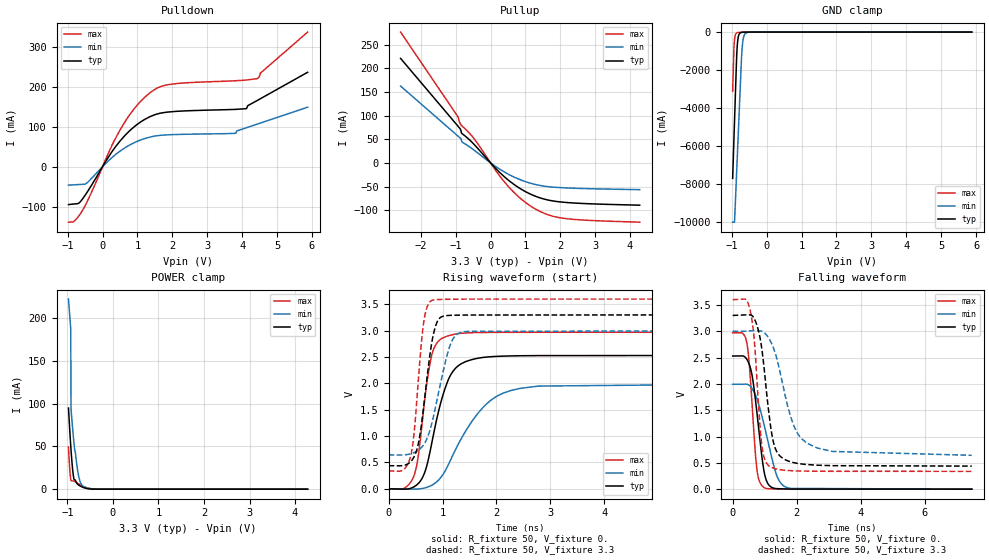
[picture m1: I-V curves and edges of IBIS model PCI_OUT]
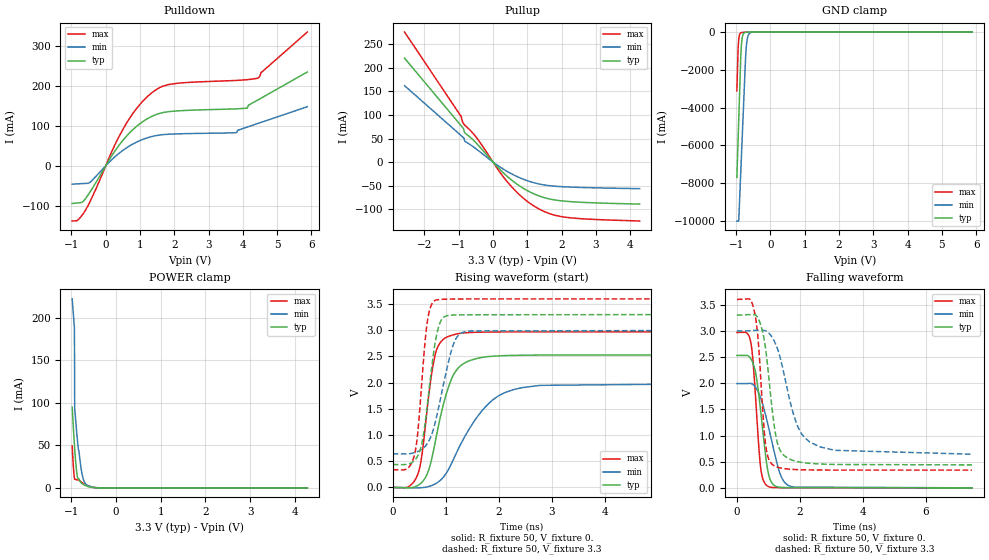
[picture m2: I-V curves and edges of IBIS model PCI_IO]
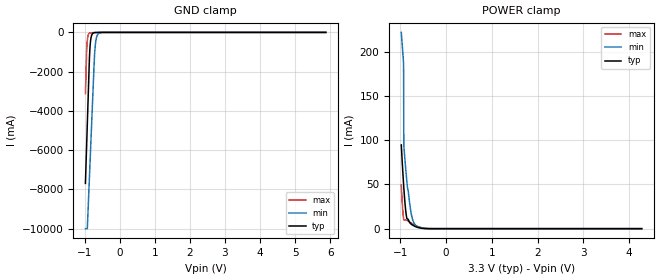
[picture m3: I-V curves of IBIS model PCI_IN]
|   IBIS Model for tsi381
[IBIS Ver]   3.2
[Disclaimer] THIS IBIS MODEL HAS BEEN CREATED BY THE SIGNAL
   INTEGRITY SOFTWARE SPICE-TO-IBIS PROCESS.
   THESE IBIS MODELS ARE PROVIDED "AS IS" WITH NO
   WARRANTY WHATSOEVER AND SIGNAL INTEGRITY SOFTWARE
   SPECIFICALLY DISCLAIMS ANY IMPLIED WARRANTIES OF
   MERCHANTABILITY, FITNESS FOR A PARTICULAR PURPOSE,
   OR AGAINST INFRINGEMENT.
[File Name]   tsi381_pbga.ibs
[File Rev]   1.4
[Date]   07/29/2009
[Notes]
   Revision History
   Rev 1.0
   - 5/30/07 Inital Release. IBIS model generated from
   SPICE model extraction. TSC
   Rev 1.3
   - 11/13/08  Updated 'model_name' definitions. IGT
   Rev 1.4
   - updated with IDT formatting
[Component] tsi381
[Manufacturer] IDT
|   typ   min   max
[Package]
R_pkg   354m   244m   481m
L_pkg   4.50nH   2.81nH   7.01nH
C_pkg   0.86pF   0.64pF   1.33pF
[Pin]  signal_name   model_name   R_pin   L_pin   C_pin
C9   GPIO[0]   NC   299.8m   3.7nh   0.83pf
A10   GPIO[1]   NC   274.4m   3.5nh   0.76pf
B10   GPIO[2]   NC   247.9m   3.3nh   0.64pf
A11   GPIO[3]   NC   287.0m   3.6nh   0.79pf
M2   JTAG_TCK   JTAG_IN   366.2m   4.4nh   0.83pf
L3   JTAG_TDI   JTAG_IN   382.4m   4.9nh   0.94pf
L1   JTAG_TDO   JTAG_OUT   371.7m   4.5nh   0.76pf
M12   JTAG_TMS   JTAG_IN   393.2m   4.5nh   0.85pf
L10   JTAG_TRSTn   JTAG_IN   410.4m   5.3nh   0.96pf
D3   PCI_AD[0]   PCI_IO   398.2m   5.4nh   0.99pf
C1   PCI_AD[1]   PCI_IO   344.1m   4.1nh   0.77pf
F4   PCI_AD[10]   PCI_IO   402.7m   5.8nh   1.06pf
G1   PCI_AD[11]   PCI_IO   310.8m   3.7nh   0.64pf
G2   PCI_AD[12]   PCI_IO   330.2m   4.0nh   0.77pf
G3   PCI_AD[13]   PCI_IO   375.2m   4.9nh   0.90pf
H1   PCI_AD[14]   PCI_IO   311.3m   3.8nh   0.65pf
H2   PCI_AD[15]   PCI_IO   355.7m   4.5nh   0.82pf
J5   PCI_AD[16]   PCI_IO   481.4m   6.8nh   1.29pf
L6   PCI_AD[17]   PCI_IO   343.6m   4.4nh   0.79pf
M6   PCI_AD[18]   PCI_IO   304.3m   3.8nh   0.66pf
K6   PCI_AD[19]   PCI_IO   371.5m   5.1nh   0.92pf
D1   PCI_AD[2]   PCI_IO   330.9m   3.9nh   0.72pf
J6   PCI_AD[20]   PCI_IO   386.3m   5.7nh   1.04pf
M7   PCI_AD[21]   PCI_IO   301.3m   3.7nh   0.65pf
L7   PCI_AD[22]   PCI_IO   326.6m   4.1nh   0.77pf
K7   PCI_AD[23]   PCI_IO   373.6m   4.9nh   0.92pf
L8   PCI_AD[24]   PCI_IO   357.1m   4.4nh   0.81pf
K8   PCI_AD[25]   PCI_IO   437.6m   5.8nh   1.12pf
M9   PCI_AD[26]   PCI_IO   323.3m   3.9nh   0.69pf
L9   PCI_AD[27]   PCI_IO   357.9m   4.5nh   0.84pf
K12   PCI_AD[28]   PCI_IO   346.8m   4.1nh   0.79pf
J11   PCI_AD[29]   PCI_IO   377.8m   4.7nh   0.93pf
D2   PCI_AD[3]   PCI_IO   353.3m   4.5nh   0.85pf
J12   PCI_AD[30]   PCI_IO   324.4m   4.0nh   0.74pf
J10   PCI_AD[31]   PCI_IO   436.5m   5.9nh   1.16pf
E1   PCI_AD[4]   PCI_IO   309.0m   3.7nh   0.67pf
E2   PCI_AD[5]   PCI_IO   352.5m   4.6nh   0.82pf
E3   PCI_AD[6]   PCI_IO   368.0m   5.0nh   0.94pf
E4   PCI_AD[7]   PCI_IO   480.4m   7.0nh   1.32pf
F2   PCI_AD[8]   PCI_IO   343.3m   4.2nh   0.79pf
F3   PCI_AD[9]   PCI_IO   363.1m   4.8nh   0.91pf
F1   PCI_CBEn[0]   PCI_IO   303.6m   3.7nh   0.65pf
H3   PCI_CBEn[1]   PCI_IO   392.2m   5.0nh   0.94pf
K5   PCI_CBEn[2]   PCI_IO   406.7m   5.4nh   1.06pf
M8   PCI_CBEn[3]   PCI_IO   309.0m   3.8nh   0.66pf
D12   PCI_CLK   PCI_IN   328.4m   3.9nh   0.67pf
H10   PCI_CLKO[0]   PCI_OUT   407.4m   5.6nh   1.09pf
C2   PCI_CLKO[1]   PCI_OUT   408.8m   5.2nh   0.95pf
K4   PCI_DEVSELn   PCI_IO   467.5m   6.4nh   1.28pf
M5   PCI_FRAMEn   PCI_IO   317.2m   3.8nh   0.68pf
G10   PCI_GNTn[0]   PCI_IO   377.6m   4.9nh   1.01pf
G9   PCI_GNTn[1]   PCI_OUT   404.4m   5.5nh   1.09pf
F11   PCI_GNTn[2]   PCI_OUT   346.6m   4.4nh   0.82pf
E11   PCI_GNTn[3]   PCI_OUT   340.9m   4.1nh   0.79pf
E12   PCI_INTAn   PCI_IN   321.7m   4.0nh   0.66pf
E9   PCI_INTBn   PCI_IN   395.4m   5.5nh   1.06pf
D11   PCI_INTCn   PCI_IN   380.1m   4.7nh   0.82pf
E10   PCI_INTDn   PCI_IN   390.8m   5.0nh   0.93pf
L5   PCI_IRDYn   PCI_IO   351.2m   4.5nh   0.87pf
M3   PCI_LOCKn   PCI_OUT   333.8m   4.2nh   0.69pf
D10   PCI_M66EN   PCI_IN   420.4m   5.6nh   0.97pf
J1   PCI_PAR   PCI_IO   328.0m   4.0nh   0.66pf
J3   PCI_PERRn   PCI_IO   436.6m   5.7nh   1.06pf
H12   PCI_PMEn   PCI_IN   326.8m   3.9nh   0.74pf
G11   PCI_REQn[0]   PCI_IO   348.8m   4.3nh   0.85pf
H9   PCI_REQn[1]   PCI_IN   420.8m   6.1nh   1.09pf
G12   PCI_REQn[2]   PCI_IN   305.3m   3.7nh   0.68pf
H11   PCI_REQn[3]   PCI_IN   335.4m   4.3nh   0.81pf
F10   PCI_RSTn   PCI_OUT   366.0m   4.9nh   0.90pf
J2   PCI_SERRn   PCI_IO   376.6m   4.8nh   0.83pf
L4   PCI_STOPn   PCI_IO   385.4m   4.9nh   0.95pf
M4   PCI_TRDYn   PCI_IO   326.3m   3.9nh   0.74pf
B12   PCIE_PERSTn   NC   347.3m   4.3nh   0.66pf
B6   PCIE_REFCLK_n   NC   339.4m   4.2nh   1.02pf
A6   PCIE_REFCLK_p   NC   341.4m   4.1nh   1.01pf
B7   PCIE_RXD_n   NC   253.1m   3.1nh   0.75pf
A8   PCIE_RXD_p   NC   266.3m   3.4nh   0.79pf
A4   PCIE_TXD_n   NC   249.7m   3.3nh   0.69pf
B5   PCIE_TXD_p   NC   244.8m   3.0nh   0.69pf
K11   PWRUP_EN_ARB   GEN33_IN   407.8m   5.1nh   1.04pf
M1   PWRUP_PLL_BYPASS   GEN33_IN   410.2m   4.8nh   0.93pf
B2   SR_CLK   NC   418.6m   5.1nh   0.96pf
C4   SR_CSn   NC   412.7m   5.5nh   1.33pf
A2   SR_DIN   NC   308.5m   3.8nh   0.87pf
A1   SR_DOUT   NC   366.1m   4.5nh   0.78pf
C8   TEST_BCE   NC   313.4m   4.3nh   0.96pf
B1   TEST_BIDR_CTL   NC   371.0m   4.4nh   0.80pf
A3   TEST_ON   NC   332.2m   4.3nh   0.93pf
M11   TEST_SPARE[0]   NC   371.4m   4.4nh   0.79pf
D8   TEST_SPARE[1]   NC   252.7m   2.8nh   0.70pf
K1   TEST_SPARE[2]   NC   349.1m   4.3nh   0.71pf
C10   VDD   POWER
D4   VDD   POWER
F6   VDD   POWER
F8   VDD   POWER
G6   VDD   POWER
G7   VDD   POWER
J9   VDD   POWER
K3   VDD   POWER
B3   VDD_PCI   POWER
B11   VDD_PCI   POWER
F9   VDD_PCI   POWER
G4   VDD_PCI   POWER
H5   VDD_PCI   POWER
H8   VDD_PCI   POWER
J7   VDD_PCI   POWER
L2   VDD_PCI   POWER
M10   VDD_PCI   POWER
A5   VDD_PCIE   POWER
A7   VDD_PCIE   POWER
D5   VDD_PCIE   POWER
E5   VDDA_PCIE   POWER
E7   VDDA_PLL   POWER
F5   VIO_PCI   POWER
G8   VIO_PCI   POWER
H6   VIO_PCI   POWER
B8   VSS   GND
B4   VSS   GND
C6   VSS   GND
C5   VSS   GND
D9   VSS   GND
D7   VSS   GND
D6   VSS   GND
E6   VSS   GND
F7   VSS   GND
G5   VSS   GND
H7   VSS   GND
H4   VSS   GND
A12   VSS_IO   GND
C11   VSS_IO   GND
C3   VSS_IO   GND
F12   VSS_IO   GND
J8   VSS_IO   GND
J4   VSS_IO   GND
K10   VSS_IO   GND
K2   VSS_IO   GND
C7   VSSA_PLL   GND
| Models and submodels in the file (6): PCI_OUT (Output), PCI_IO (I/O), PCI_IN (Input), JTAG_IN (Input), JTAG_OUT (Output), GEN33_IN (Input)
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[Model]   PCI_OUT
Model_type  Output
C_comp 4.536p 4.202p 4.874p
Polarity   Non-Inverting
Enable   Active-High
Vmeas =   1.32V
Cref =   10pF
Rref =   50
Vref=   0.0V
[Temperature Range]   27.0   125.0   -40.0
[Voltage Range] 3.3 3. 3.6
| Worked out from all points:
|   slope of the pulldown table from 0 to 0.495 V, typ, clamps not added: 7.81 ohm
|   slope of the pullup table from 0 to 0.495 V, typ, clamps not added: 13.9 ohm
|   GND clamp passes 1 mA (typ) near -0.58 V on its own axis
|   POWER clamp passes 1 mA (typ) near -0.59 V on its own axis
|   rising waveform, R_fixture 50, V_fixture 0.: 20-80 % time 365ps typ, 723ps min, 222ps max; typ from 0 V to 2.53 V
|   rising waveform, R_fixture 50, V_fixture 3.3: 20-80 % time 214ps typ, 317ps min, 159ps max; typ from 0.438 V to 3.3 V
|   falling waveform, R_fixture 50, V_fixture 0.: 20-80 % time 295ps typ, 484ps min, 203ps max; typ from 2.53 V to 0 V
|   falling waveform, R_fixture 50, V_fixture 3.3: 20-80 % time 338ps typ, 623ps min, 226ps max; typ from 3.3 V to 0.438 V
[Pulldown]
-976.9mV  -94.66mA   -46.06mA   -138.7mA
-817.5mV  -93.23mA   -45.29mA   -136.5mA
-595.7mV  -83.14mA   -44.21mA   -112.2mA
-429.3mV  -61.97mA   -39.17mA   -84.92mA
492.7mV   63.11mA    38.33mA    90.31mA
936.3mV   101.8mA    61.1mA     147.9mA
1.352V    124.6mA    73.73mA    184.1mA
1.851V    136.3mA    79.48mA    204.5mA
3.82V     143.1mA    83.35mA    214.6mA
4.125V    144.9mA    97.25mA    216.4mA
4.43V     165.1mA    106.2mA    220mA
5.879V    235.8mA    148.6mA    336.1mA
[Pullup]
-2.579V   220.8mA    162.3mA    276.3mA
-929mV    77.21mA    56.24mA    96.97mA
-887.4mV  73.58mA    53.57mA    85.73mA
-838.9mV  65.18mA    49.35mA    79.56mA
-818.1mV  61.78mA    43.99mA    77.84mA
-471.5mV  38.99mA    26.83mA    51.07mA
277.2mV   -21.28mA   -14.01mA   -29.14mA
623.8mV   -42.97mA   -28.22mA   -58.92mA
942.6mV   -58.4mA    -38.19mA   -80.33mA
1.442V    -74.52mA   -48.11mA   -103.5mA
1.969V    -82.31mA   -52.22mA   -115.7mA
4.277V    -89.5mA    -56.68mA   -125.4mA
[GND Clamp]
-976.9mV  -7.694A    -10A       -3.11A
-940.4mV  -5.645A    -10A       -848.5mA
-923.3mV  -4.682A    -10A       -400.9mA
-899.6mV  -3.359A    -8.991A    -148.3mA
-863.2mV  -1.353A    -7.407A    -43.18mA
-837.4mV  -553.5mA   -6.29A     -25.04mA
-794.5mV  -126.9mA   -4.431A    -15.74mA
-727.9mV  -18.49mA   -1.562A    -9.993mA
-708.6mV  -11.57mA   -935.5mA   -8.672mA
-670mV    -5.111mA   -330.6mA   -6.269mA
-603.5mV  -1.592mA   -60.06mA   -2.971mA
5.879V    0A         0A         0A
[Power Clamp]
-976.9mV  94.83mA    222.1mA    49.21mA
-949.3mV  68.95mA    202.6mA    23.59mA
-927.1mV  50.38mA    187.5mA    11.34mA
-921.6mV  46.09mA    93.87mA    10.01mA
-888.4mV  24.44mA    72.65mA    9.649mA
-855.2mV  11.42mA    53.18mA    9.29mA
-783.3mV  6.267mA    24.59mA    7.167mA
-750.1mV  4.693mA    14.57mA    6.03mA
-705.8mV  3.303mA    6.993mA    4.715mA
-656.1mV  2.103mA    3.495mA    3.408mA
-357.3mV  8.391uA    72.94uA    14.41uA
4.277V    0A         0A         0A
[Ramp]
dV/dt_r 1.518/365.23p 1.196/721.023p 1.782/221.8p
dV/dt_f 1.717/337.435p 1.415/622.991p 1.957/226.082p
[Rising Waveform]
R_fixture = 50
V_fixture = 0.
0s        0V         0V         0V
470ps     37.05mV    -6.726mV   246.6mV
550ps     99.96mV    -3.323mV   620.7mV
650ps     259.3mV    11.36mV    1.507V
800ps     863.9mV    67.25mV    2.539V
1.05ns    1.912V     341.7mV    2.883V
1.27ns    2.315V     802.2mV    2.942V
1.67ns    2.48V      1.449V     2.965V
2.28ns    2.522V     1.869V     2.969V
7.47ns    2.529V     1.993V     2.97V
[Rising Waveform]
R_fixture = 50
V_fixture = 3.3
V_fixture_min = 3.
V_fixture_max = 3.6
0s        438.2mV    642.1mV    338.6mV
410ps     515.4mV    664.5mV    626mV
470ps     601.9mV    685.9mV    1.029V
550ps     848.7mV    731.3mV    2.042V
650ps     1.557V     836.6mV    3.151V
800ps     2.767V     1.238V     3.573V
930ps     3.219V     1.841V     3.591V
1.13ns    3.29V      2.691V     3.596V
1.35ns    3.296V     2.969V     3.599V
7.47ns    3.3V       3V         3.6V
[Falling Waveform]
R_fixture = 50
V_fixture = 0.
0s        2.529V     1.993V     2.97V
440ps     2.469V     1.994V     2.787V
510ps     2.384V     1.976V     2.438V
600ps     2.182V     1.917V     1.677V
760ps     1.445V     1.712V     366.7mV
980ps     340.4mV    1.227V     32.06mV
1.12ns    87.95mV    862.5mV    8.858mV
1.38ns    10.32mV    256.9mV    3.596mV
1.74ns    3.211mV    22.96mV    1.388mV
7.47ns    1.068uV    15.07uV    0V
[Falling Waveform]
R_fixture = 50
V_fixture = 3.3
V_fixture_min = 3.
V_fixture_max = 3.6
0s        3.3V       3V         3.6V
420ps     3.311V     3.001V     3.601V
560ps     3.308V     3.009V     3.356V
680ps     3.232V     3.01V      2.799V
910ps     2.668V     3V         845.2mV
1.15ns    1.357V     2.845V     435.1mV
1.44ns    655.6mV    2.332V     374.1mV
1.88ns    507.9mV    1.256V     349.5mV
2.32ns    467.9mV    874.5mV    342.5mV
7.47ns    438.2mV    643.1mV    338.6mV
[Model]   PCI_IO
Model_type  I/O
C_comp 4.536p 4.202p 4.874p
Polarity   Non-Inverting
Enable   Active-High
Vinl =   0.80V
Vinh =   2.00V
Vmeas =   1.32V
Cref =   10pF
Rref =   50
Vref=   0.0V
[Temperature Range]   27.0   125.0   -40.0
[Voltage Range] 3.3 3. 3.6
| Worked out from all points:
|   slope of the pulldown table from 0 to 0.495 V, typ, clamps not added: 7.81 ohm
|   slope of the pullup table from 0 to 0.495 V, typ, clamps not added: 13.9 ohm
|   GND clamp passes 1 mA (typ) near -0.58 V on its own axis
|   POWER clamp passes 1 mA (typ) near -0.59 V on its own axis
|   rising waveform, R_fixture 50, V_fixture 0.: 20-80 % time 365ps typ, 723ps min, 222ps max; typ from 0 V to 2.53 V
|   rising waveform, R_fixture 50, V_fixture 3.3: 20-80 % time 214ps typ, 317ps min, 159ps max; typ from 0.438 V to 3.3 V
|   falling waveform, R_fixture 50, V_fixture 0.: 20-80 % time 295ps typ, 484ps min, 203ps max; typ from 2.53 V to 0 V
|   falling waveform, R_fixture 50, V_fixture 3.3: 20-80 % time 338ps typ, 623ps min, 226ps max; typ from 3.3 V to 0.438 V
[Pulldown]
-976.9mV  -94.66mA   -46.06mA   -138.7mA
-817.5mV  -93.23mA   -45.29mA   -136.5mA
-595.7mV  -83.14mA   -44.21mA   -112.2mA
-429.3mV  -61.97mA   -39.17mA   -84.92mA
492.7mV   63.11mA    38.33mA    90.31mA
936.3mV   101.8mA    61.1mA     147.9mA
1.352V    124.6mA    73.73mA    184.1mA
1.851V    136.3mA    79.48mA    204.5mA
3.82V     143.1mA    83.35mA    214.6mA
4.125V    144.9mA    97.25mA    216.4mA
4.43V     165.1mA    106.2mA    220mA
5.879V    235.8mA    148.6mA    336.1mA
[Pullup]
-2.579V   220.8mA    162.3mA    276.3mA
-929mV    77.21mA    56.24mA    96.97mA
-887.4mV  73.58mA    53.57mA    85.73mA
-838.9mV  65.18mA    49.35mA    79.56mA
-818.1mV  61.78mA    43.99mA    77.84mA
-471.5mV  38.99mA    26.83mA    51.07mA
277.2mV   -21.28mA   -14.01mA   -29.14mA
623.8mV   -42.97mA   -28.22mA   -58.92mA
942.6mV   -58.4mA    -38.19mA   -80.33mA
1.442V    -74.52mA   -48.11mA   -103.5mA
1.969V    -82.31mA   -52.22mA   -115.7mA
4.277V    -89.5mA    -56.68mA   -125.4mA
[GND Clamp]
-976.9mV  -7.694A    -10A       -3.11A
-940.4mV  -5.645A    -10A       -848.5mA
-923.3mV  -4.682A    -10A       -400.9mA
-899.6mV  -3.359A    -8.991A    -148.3mA
-863.2mV  -1.353A    -7.407A    -43.18mA
-837.4mV  -553.5mA   -6.29A     -25.04mA
-794.5mV  -126.9mA   -4.431A    -15.74mA
-727.9mV  -18.49mA   -1.562A    -9.993mA
-708.6mV  -11.57mA   -935.5mA   -8.672mA
-670mV    -5.111mA   -330.6mA   -6.269mA
-603.5mV  -1.592mA   -60.06mA   -2.971mA
5.879V    0A         0A         0A
[Power Clamp]
-976.9mV  94.83mA    222.1mA    49.21mA
-949.3mV  68.95mA    202.6mA    23.59mA
-927.1mV  50.38mA    187.5mA    11.34mA
-921.6mV  46.09mA    93.87mA    10.01mA
-888.4mV  24.44mA    72.65mA    9.649mA
-855.2mV  11.42mA    53.18mA    9.29mA
-783.3mV  6.267mA    24.59mA    7.167mA
-750.1mV  4.693mA    14.57mA    6.03mA
-705.8mV  3.303mA    6.993mA    4.715mA
-656.1mV  2.103mA    3.495mA    3.408mA
-357.3mV  8.391uA    72.94uA    14.41uA
4.277V    0A         0A         0A
[Ramp]
dV/dt_r 1.518/365.23p 1.196/721.023p 1.782/221.8p
dV/dt_f 1.717/337.435p 1.415/622.991p 1.957/226.082p
[Rising Waveform]
R_fixture = 50
V_fixture = 0.
0s        0V         0V         0V
470ps     37.05mV    -6.726mV   246.6mV
550ps     99.96mV    -3.323mV   620.7mV
650ps     259.3mV    11.36mV    1.507V
800ps     863.9mV    67.25mV    2.539V
1.05ns    1.912V     341.7mV    2.883V
1.27ns    2.315V     802.2mV    2.942V
1.67ns    2.48V      1.449V     2.965V
2.28ns    2.522V     1.869V     2.969V
7.47ns    2.529V     1.993V     2.97V
[Rising Waveform]
R_fixture = 50
V_fixture = 3.3
V_fixture_min = 3.
V_fixture_max = 3.6
0s        438.2mV    642.1mV    338.6mV
410ps     515.4mV    664.5mV    626mV
470ps     601.9mV    685.9mV    1.029V
550ps     848.7mV    731.3mV    2.042V
650ps     1.557V     836.6mV    3.151V
800ps     2.767V     1.238V     3.573V
930ps     3.219V     1.841V     3.591V
1.13ns    3.29V      2.691V     3.596V
1.35ns    3.296V     2.969V     3.599V
7.47ns    3.3V       3V         3.6V
[Falling Waveform]
R_fixture = 50
V_fixture = 0.
0s        2.529V     1.993V     2.97V
440ps     2.469V     1.994V     2.787V
510ps     2.384V     1.976V     2.438V
600ps     2.182V     1.917V     1.677V
760ps     1.445V     1.712V     366.7mV
980ps     340.4mV    1.227V     32.06mV
1.12ns    87.95mV    862.5mV    8.858mV
1.38ns    10.32mV    256.9mV    3.596mV
1.74ns    3.211mV    22.96mV    1.388mV
7.47ns    1.068uV    15.07uV    0V
[Falling Waveform]
R_fixture = 50
V_fixture = 3.3
V_fixture_min = 3.
V_fixture_max = 3.6
0s        3.3V       3V         3.6V
420ps     3.311V     3.001V     3.601V
560ps     3.308V     3.009V     3.356V
680ps     3.232V     3.01V      2.799V
910ps     2.668V     3V         845.2mV
1.15ns    1.357V     2.845V     435.1mV
1.44ns    655.6mV    2.332V     374.1mV
1.88ns    507.9mV    1.256V     349.5mV
2.32ns    467.9mV    874.5mV    342.5mV
7.47ns    438.2mV    643.1mV    338.6mV
|   MODEL PCI_IN
[Model]   PCI_IN
Model_type  Input
C_comp 4.536p 4.202p 4.874p
Polarity   Non-Inverting
Enable   Active-High
Vinl =   0.80V
Vinh =   2.00V
[Temperature Range]   27.0   125.0   -40.0
[POWER Clamp Reference]   3.30V   3.00V   3.60V
[GND Clamp Reference]   0.00V   0.00V   0.00V
[Voltage Range] 3.3 3. 3.6
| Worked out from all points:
|   GND clamp passes 1 mA (typ) near -0.58 V on its own axis
|   POWER clamp passes 1 mA (typ) near -0.59 V on its own axis
[GND Clamp]
-976.9mV  -7.694A    -10A       -3.11A
-940.4mV  -5.645A    -10A       -848.5mA
-923.3mV  -4.682A    -10A       -400.9mA
-899.6mV  -3.359A    -8.991A    -148.3mA
-863.2mV  -1.353A    -7.407A    -43.18mA
-837.4mV  -553.5mA   -6.29A     -25.04mA
-794.5mV  -126.9mA   -4.431A    -15.74mA
-727.9mV  -18.49mA   -1.562A    -9.993mA
-708.6mV  -11.57mA   -935.5mA   -8.672mA
-670mV    -5.111mA   -330.6mA   -6.269mA
-603.5mV  -1.592mA   -60.06mA   -2.971mA
5.879V    0A         0A         0A
[Power Clamp]
-976.9mV  94.83mA    222.1mA    49.21mA
-949.3mV  68.95mA    202.6mA    23.59mA
-927.1mV  50.38mA    187.5mA    11.34mA
-921.6mV  46.09mA    93.87mA    10.01mA
-888.4mV  24.44mA    72.65mA    9.649mA
-855.2mV  11.42mA    53.18mA    9.29mA
-783.3mV  6.267mA    24.59mA    7.167mA
-750.1mV  4.693mA    14.57mA    6.03mA
-705.8mV  3.303mA    6.993mA    4.715mA
-656.1mV  2.103mA    3.495mA    3.408mA
-357.3mV  8.391uA    72.94uA    14.41uA
4.277V    0A         0A         0A
